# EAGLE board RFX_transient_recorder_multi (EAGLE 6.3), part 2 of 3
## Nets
+2.5V: C18.+ C22.2 C23.2 U5.5 U6.2 U6.44
+2.5V1: C64.+ C65.2 C66.2 U1.2 U1.44 U21.5
+2.5V2: C106.+ C107.2 C108.2 U25.2 U25.44 U33.5
+2.5V3: C148.+ C149.2 C150.2 U37.2 U37.44 U45.5
+2.5V_DIG: C29.2 C30.+ U6.19 U8.5
+2.5V_DIG1: C69.+ C70.2 U1.19 U22.5
+2.5V_DIG2: C111.+ C112.2 U25.19 U34.5
+2.5V_DIG3: C153.+ C154.2 U37.19 U46.5
+3.0V: C14.2 C15.2 C16.+ IC2.8 U4.5 U$1.5 U$1.6 U$1.7 U$1.8
+3.0V1: C50.2 C52.+ C71.2 IC4.8 U20.5 U$2.5 U$2.6 U$2.7 U$2.8
+3.0V2: C92.2 C94.+ C113.2 IC6.8 U32.5 U$3.5 U$3.6 U$3.7 U$3.8
+3.0V3: C134.2 C136.+ C155.2 IC8.8 U44.5 U$4.5 U$4.6 U$4.7 U$4.8
+3V1: C67.+ C68.2 C73.2 C77.2 C78.2 U1.3 U1.4 U1.6 U1.16 U1.18 U2.7 U2.8 U3.1 U16.8 U23.5
+3V2: C109.+ C110.2 C115.2 C119.2 C120.2 U25.3 U25.4 U25.6 U25.16 U25.18 U26.7 U26.8 U27.1 U28.8 U35.5
+3V3: C27.+ C28.2 C32.2 C33.2 C34.2 U6.3 U6.4 U6.6 U6.16 U6.18 U7.5 U9.7 U9.8 U11.1 U12.8
+3V3_ISOL: C35.1 C36.1 C38.+ C41.2 C42.2 R26.2 U11.8 U12.1 U15.4 U15.8
+3V3_ISOL1: C75.1 C76.1 C79.2 C80.2 C84.+ R53.2 U3.8 U16.1 U17.4 U17.8
+3V3_ISOL2: C117.1 C118.1 C121.2 C122.2 C126.+ R81.2 U27.8 U28.1 U29.4 U29.8
+3V3_ISOL3: C159.1 C160.1 C163.2 C164.2 C168.+ R109.2 U39.8 U40.1 U41.4 U41.8
+3V4: C151.+ C152.2 C157.2 C161.2 C162.2 U37.3 U37.4 U37.6 U37.16 U37.18 U38.7 U38.8 U39.1 U40.8 U47.5
+5V_ISOL: C37.+ U10.P$1 U13.1 U13.3
+5V_ISOL1: C83.+ U19.1 U19.3 U24.P$1
+5V_ISOL2: C125.+ U31.1 U31.3 U36.P$1
+5V_ISOL3: C167.+ U43.1 U43.3 U48.P$1
-2.0V_NEG: C4.1 C5.- C6.2 C7.2 IC1.5 IC2.4 R5.2 U$1.13 U$1.14 U$1.15 U$1.16
-2.0V_NEG1: C51.2 C53.- C58.1 C60.2 IC3.5 IC4.4 R33.2 U$2.13 U$2.14 U$2.15 U$2.16
-2.0V_NEG2: C93.2 C95.- C100.1 C102.2 IC5.5 IC6.4 R61.2 U$3.13 U$3.14 U$3.15 U$3.16
-2.0V_NEG3: C135.2 C137.- C142.1 C144.2 IC7.5 IC8.4 R89.2 U$4.13 U$4.14 U$4.15 U$4.16
AGND: C4.2 C5.+ C6.1 C7.1 C11.1 C12.1 C13.2 C14.1 C15.1 C16.- C17.2 C18.- C19.2 C20.- C21.2 C22.1 C23.1 C43.1 IC1.1 IC2.3 R4.2 R17..2 R28.2 U4.2 U5.2 U6.1 U6.36 U6.38 U6.41 U6.42 U6.47 U6.48 X1.1 X1.2 X1.5 X1.6 X2.1 X2.2 X2.5 X2.6 X3.1 X3.2 X3.5 X3.6 X4.1 X4.2 X4.5 X4.6
AGND1: C47.1 C48.1 C49.1 C50.1 C51.1 C52.- C53.+ C54.2 C55.2 C58.2 C60.1 C61.2 C62.- C63.2 C64.- C65.1 C66.1 C71.1 IC3.1 IC4.3 R17.1.2 R32.2 R55.2 U1.1 U1.36 U1.38 U1.41 U1.42 U1.47 U1.48 U20.2 U21.2 X6.1 X6.2 X6.5 X6.6
AGND2: C89.1 C90.1 C91.1 C92.1 C93.1 C94.- C95.+ C96.2 C97.2 C100.2 C102.1 C103.2 C104.- C105.2 C106.- C107.1 C108.1 C113.1 IC5.1 IC6.3 R17.2.2 R60.2 R83.2 U25.1 U25.36 U25.38 U25.41 U25.42 U25.47 U25.48 U32.2 U33.2 X8.1 X8.2 X8.5 X8.6
AGND3: C131.1 C132.1 C133.1 C134.1 C135.1 C136.- C137.+ C138.2 C139.2 C142.2 C144.1 C145.2 C146.- C147.2 C148.- C149.1 C150.1 C155.1 IC7.1 IC8.3 R17.3.2 R88.2 R111.2 U37.1 U37.36 U37.38 U37.41 U37.42 U37.47 U37.48 U44.2 U45.2 X10.1 X10.2 X10.5 X10.6
GNDI: C2..+ C24.1 C25.- C26.2 C27.- C28.1 C29.1 C30.- C31.2 C32.1 C33.1 C34.1 R17..1 R22.1 U6.5 U6.7 U6.13 U6.14 U6.15 U6.17 U6.20 U6.30 U6.31 U6.32 U6.33 U7.2 U8.2 U9.4 U10.P$5 U11.4 U12.5
GNDI1: C2.1.+ C56.2 C57.2 C59.- C67.- C68.1 C69.- C70.1 C73.1 C74.1 C77.1 C78.1 R17.1.1 R56.1 U1.5 U1.7 U1.13 U1.14 U1.15 U1.17 U1.20 U1.30 U1.31 U1.32 U1.33 U2.4 U3.4 U16.5 U22.2 U23.2 U24.P$5
GNDI2: C2.2.+ C98.2 C99.2 C101.- C109.- C110.1 C111.- C112.1 C115.1 C116.1 C119.1 C120.1 R17.2.1 R84.1 U25.5 U25.7 U25.13 U25.14 U25.15 U25.17 U25.20 U25.30 U25.31 U25.32 U25.33 U26.4 U27.4 U28.5 U34.2 U35.2 U36.P$5
GNDI3: C2.3.+ C140.2 C141.2 C143.- C151.- C152.1 C153.- C154.1 C157.1 C158.1 C161.1 C162.1 R17.3.1 R112.1 U37.5 U37.7 U37.13 U37.14 U37.15 U37.17 U37.20 U37.30 U37.31 U37.32 U37.33 U38.4 U39.4 U40.5 U46.2 U47.2 U48.P$5
ISOL_GND: C35.2 C36.2 C37.- C38.- C39.1 C40.1 C41.1 C42.1 R25.2 U10.P$2 U11.5 U12.4 U13.2 U14.4 U15.1 U15.2 U15.3 U15.6 U15.10
ISOL_GND1: C75.2 C76.2 C79.1 C80.1 C81.1 C82.1 C83.- C84.- R54.2 U3.5 U16.4 U17.1 U17.2 U17.3 U17.6 U17.10 U18.4 U19.2 U24.P$2
ISOL_GND2: C117.2 C118.2 C121.1 C122.1 C123.1 C124.1 C125.- C126.- R82.2 U27.5 U28.4 U29.1 U29.2 U29.3 U29.6 U29.10 U30.4 U31.2 U36.P$2
ISOL_GND3: C159.2 C160.2 C163.1 C164.1 C165.1 C166.1 C167.- C168.- R110.2 U39.5 U40.4 U41.1 U41.2 U41.3 U41.6 U41.10 U42.4 U43.2 U48.P$2
N$1: C3.1 L1.2 R6.2
N$2: C1.1 L1.1 R2.1
N$3: C3.2 L2.2 R7.2
N$4: C1.2 L2.1 R3.1
N$5: C9.1 R6.1 R9.1 R11.2 U$1.11
N$6: C10.1 R7.1 R8.1 R12.2 U$1.2
N$7: R20.2 U9.1
N$8: R1.2 R2.2 X1.3
N$9: R1.1 R3.2 X1.4
N$10: C9.2 R11.1 R14.2 U$1.10
N$11: C10.2 R12.1 R15.2 U$1.3
N$12: C11.2 R14.1 U6.39
N$13: C12.2 R15.1 U6.43
N$14: R28.1
N$15: R22.2
N$16: C2..- IC1.2 IC1.3 U10.P$7 X1.9 X1.10
N$17: C17.1 U4.4
N$18: C25.+ U4.1 U4.3 U5.1 U5.3 U7.1 U7.3 U8.1 U8.3 U10.P$6 X1.7 X1.8
N$19: X2.3
N$20: C19.1 U5.4
N$21: X2.4
N$22: X2.9 X2.10 X3.9 X3.10 X4.10
N$23: C31.1 U8.4
N$24: X2.7 X2.8 X3.7 X3.8 X4.7 X4.8
N$25: X3.3
N$26: C26.1 U7.4
N$27: IC1.4 R4.1 R5.1
N$28: C43.2 IC2.6 IC2.7 U$1.4 U$1.9
N$29: X3.4
N$30: C13.1 IC2.5 R13.1 R16.2
N$31: R20.1 U6.22
N$32: C20.+ R16.1 U6.37
N$33: C21.1 U6.46
N$34: U15.11 X5.1
N$35: U15.12 X5.2
N$36: R19.1 U6.23
N$37: R18.2 R19.2 U9.6
N$38: R18.1 U6.29
N$39: U9.2 U9.3
N$40: C8.1 IC2.1 R8.2 R9.2 R10.2
N$41: C8.2 IC2.2 R10.1 R13.2
N$42: U9.5 U11.2
N$43: R21.1 U6.21
N$44: R21.2 U11.3
N$45: C24.2 R17.2 U6.35
N$46: R17.1 U12.6
N$47: U6.34 U12.7
N$48: X4.3
N$49: X4.4
N$50: R27.1 U12.3 U14.1
N$51: R24.2 U15.5
N$52: R23.2 U15.7
N$53: R24.1 U11.7
N$54: R23.1 U11.6
N$55: U15.13 X5.3
N$56: R27.2 U15.9
N$57: R26.1 U12.2 X5.8
N$58: U15.14 X5.4
N$59: U14.2 U14.3
N$60: R25.1 U14.6 X5.7
N$61: U10.P$14 U14.5
N$62: C40.2 U13.5 U14.7 U14.8
N$63: U15.15 X5.5
N$64: C39.2 U13.4
N$65: U15.16 X5.6
N$66: C44.1 L3.2 R34.2
N$67: C2.1 L3.1 R30.1
N$68: C44.2 L4.2 R35.2
N$69: C2.2 L4.1 R31.1
N$70: C45.1 R34.1 R37.1 R38.2 U$2.11
N$71: C46.1 R35.1 R36.1 R39.2 U$2.2
N$72: R29.2 R30.2 X6.3
N$73: R29.1 R31.2 X6.4
N$74: C45.2 R38.1 R40.2 U$2.10
N$75: C46.2 R39.1 R41.2 U$2.3
N$76: C47.2 R40.1 U1.39
N$77: C48.2 R41.1 U1.43
N$78: IC3.4 R32.1 R33.1
N$79: C49.2 IC4.6 IC4.7 U$2.4 U$2.9
N$80: C61.1 IC4.5 R42.2 R43.1
N$81: C62.+ R42.1 U1.37
N$82: C63.1 U1.46
N$83: C72.1 IC4.1 R36.2 R37.2 R44.2
N$84: C72.2 IC4.2 R43.2 R44.1
N$85: R45.2 U2.1
N$86: R45.1 U1.22
N$87: R46.1 U1.23
N$88: R46.2 R47.2 U2.6
N$89: R47.1 U1.29
N$90: U2.2 U2.3
N$91: U2.5 U3.2
N$92: R48.1 U1.21
N$93: R48.2 U3.3
N$94: C74.2 R49.2 U1.35
N$95: R49.1 U16.6
N$96: U1.34 U16.7
N$97: R50.2 U17.5
N$98: R51.2 U17.7
N$99: R50.1 U3.7
N$100: R51.1 U3.6
N$101: R52.2 U17.9
N$102: R52.1 U16.3 U18.1
N$103: R53.1 U16.2 X7.8
N$104: U18.2 U18.3
N$105: R54.1 U18.6 X7.7
N$106: C81.2 U18.7 U18.8 U19.5
N$107: C82.2 U19.4
N$108: C54.1 U20.4
N$109: C55.1 U21.4
N$110: C56.1 U22.4
N$111: C57.1 U23.4
N$112: U18.5 U24.P$14
N$113: R55.1
N$114: R56.2
N$115: C2.1.- IC3.2 IC3.3 U24.P$7 X6.9 X6.10
N$116: C59.+ U20.1 U20.3 U21.1 U21.3 U22.1 U22.3 U23.1 U23.3 U24.P$6 X6.7 X6.8
N$117: U17.11 X7.1
N$118: U17.12 X7.2
N$119: U17.13 X7.3
N$120: U17.14 X7.4
N$121: U17.15 X7.5
N$122: U17.16 X7.6
N$123: C86.1 L5.2 R62.2
N$124: C85.1 L5.1 R58.1
N$125: C86.2 L6.2 R63.2
N$126: C85.2 L6.1 R59.1
N$127: C87.1 R62.1 R65.1 R66.2 U$3.11
N$128: C88.1 R63.1 R64.1 R67.2 U$3.2
N$129: R57.2 R58.2 X8.3
N$130: R57.1 R59.2 X8.4
N$131: C87.2 R66.1 R68.2 U$3.10
N$132: C88.2 R67.1 R69.2 U$3.3
N$133: C89.2 R68.1 U25.39
N$134: C90.2 R69.1 U25.43
N$135: IC5.4 R60.1 R61.1
N$136: C91.2 IC6.6 IC6.7 U$3.4 U$3.9
N$137: C103.1 IC6.5 R70.2 R71.1
N$138: C104.+ R70.1 U25.37
N$139: C105.1 U25.46
N$140: C114.1 IC6.1 R64.2 R65.2 R72.2
N$141: C114.2 IC6.2 R71.2 R72.1
N$142: R73.2 U26.1
N$143: R73.1 U25.22
N$144: R74.1 U25.23
N$145: R74.2 R75.2 U26.6
N$146: R75.1 U25.29
N$147: U26.2 U26.3
N$148: U26.5 U27.2
N$149: R76.1 U25.21
N$150: R76.2 U27.3
N$151: C116.2 R77.2 U25.35
N$152: R77.1 U28.6
N$153: U25.34 U28.7
N$154: R78.2 U29.5
N$155: R79.2 U29.7
N$156: R78.1 U27.7
N$157: R79.1 U27.6
N$158: R80.2 U29.9
N$159: R80.1 U28.3 U30.1
N$160: R81.1 U28.2 X9.8
N$161: U30.2 U30.3
N$162: R82.1 U30.6 X9.7
N$163: C123.2 U30.7 U30.8 U31.5
N$164: C124.2 U31.4
N$165: C96.1 U32.4
N$166: C97.1 U33.4
N$167: C98.1 U34.4
N$168: C99.1 U35.4
N$169: U30.5 U36.P$14
N$170: R83.1
N$171: R84.2
N$172: C2.2.- IC5.2 IC5.3 U36.P$7 X8.9 X8.10
N$173: C101.+ U32.1 U32.3 U33.1 U33.3 U34.1 U34.3 U35.1 U35.3 U36.P$6 X8.7 X8.8
N$174: U29.11 X9.1
N$175: U29.12 X9.2
N$176: U29.13 X9.3
N$177: U29.14 X9.4
N$178: U29.15 X9.5
N$179: U29.16 X9.6
N$180: C128.1 L7.2 R90.2
N$181: C127.1 L7.1 R86.1
N$182: C128.2 L8.2 R91.2
N$183: C127.2 L8.1 R87.1
N$184: C129.1 R90.1 R93.1 R94.2 U$4.11
N$185: C130.1 R91.1 R92.1 R95.2 U$4.2
N$186: R85.2 R86.2 X10.3
N$187: R85.1 R87.2 X10.4
N$188: C129.2 R94.1 R96.2 U$4.10
N$189: C130.2 R95.1 R97.2 U$4.3
N$190: C131.2 R96.1 U37.39
N$191: C132.2 R97.1 U37.43
N$192: IC7.4 R88.1 R89.1
N$193: C133.2 IC8.6 IC8.7 U$4.4 U$4.9
N$194: C145.1 IC8.5 R98.2 R99.1
N$195: C146.+ R98.1 U37.37
N$196: C147.1 U37.46
N$197: C156.1 IC8.1 R92.2 R93.2 R100.2
N$198: C156.2 IC8.2 R99.2 R100.1
N$199: R101.2 U38.1
N$200: R101.1 U37.22
N$201: R102.1 U37.23
N$202: R102.2 R103.2 U38.6
N$203: R103.1 U37.29
N$204: U38.2 U38.3
N$205: U38.5 U39.2
N$206: R104.1 U37.21
N$207: R104.2 U39.3
N$208: C158.2 R105.2 U37.35
N$209: R105.1 U40.6
N$210: U37.34 U40.7
N$211: R106.2 U41.5
N$212: R107.2 U41.7
N$213: R106.1 U39.7
N$214: R107.1 U39.6
N$215: R108.2 U41.9
N$216: R108.1 U40.3 U42.1
N$217: R109.1 U40.2 X11.8
N$218: U42.2 U42.3
N$219: R110.1 U42.6 X11.7
N$220: C165.2 U42.7 U42.8 U43.5
N$221: C166.2 U43.4
N$222: C138.1 U44.4
N$223: C139.1 U45.4
N$224: C140.1 U46.4
N$225: C141.1 U47.4
N$226: U42.5 U48.P$14
N$227: R111.1
N$228: R112.2
N$229: C2.3.- IC7.2 IC7.3 U48.P$7 X10.9 X10.10
N$230: C143.+ U44.1 U44.3 U45.1 U45.3 U46.1 U46.3 U47.1 U47.3 U48.P$6 X10.7 X10.8
N$231: U41.11 X11.1
N$232: U41.12 X11.2
N$233: U41.13 X11.3
N$234: U41.14 X11.4
N$235: U41.15 X11.5
N$236: U41.16 X11.6

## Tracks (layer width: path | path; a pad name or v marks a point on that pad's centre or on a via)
+2.5V
  Top 0.254: 55.9,84.53 56.5,84.53 56.5,83.93 C23.2 56.5,83.73 56.5,81.33 C22.2 56.6,81.23 57.4,80.43 57.4,74.33 | 55.9,84.53 51.1,84.53 U6.44 | 55.9,84.53 55.9,86.83 55.7,87.03 55.7,88.83 49.5,88.83 49.3,88.63 49.3,87.93 U6.2 | 57.4,74.33 61.4,74.33 62.2,75.13 62.2,76.53 U5.5 | C18.+ 43,76.13 44.9,74.23 57.3,74.23 57.3,74.33 57.4,74.33
+2.5V1
  Top 0.254: 55.9,12.14 56.5,12.14 56.5,11.54 C66.2 56.5,11.34 56.5,8.94 C65.2 56.6,8.84 57.4,8.04 57.4,1.94 | 55.9,12.14 51.1,12.14 U1.44 | 55.9,12.14 55.9,14.44 55.7,14.64 55.7,16.44 49.5,16.44 49.3,16.24 49.3,15.54 U1.2 | 57.4,1.94 61.4,1.94 62.2,2.74 62.2,4.14 U21.5 | C64.+ 43,3.74 44.9,1.84 57.3,1.84 57.3,1.94 57.4,1.94
+2.5V2
  Top 0.254: 55.9,60.4 56.5,60.4 56.5,59.8 C108.2 56.5,59.6 56.5,57.2 C107.2 56.6,57.1 57.4,56.3 57.4,50.2 | 55.9,60.4 51.1,60.4 U25.44 | 55.9,60.4 55.9,62.7 55.7,62.9 55.7,64.7 49.5,64.7 49.3,64.5 49.3,63.8 U25.2 | 57.4,50.2 61.4,50.2 62.2,51 62.2,52.4 U33.5 | C106.+ 43,52 44.9,50.1 57.3,50.1 57.3,50.2 57.4,50.2
+2.5V3
  Top 0.254: 55.9,36.27 56.5,36.27 56.5,35.67 C150.2 56.5,35.47 56.5,33.07 C149.2 56.6,32.97 57.4,32.17 57.4,26.07 | 55.9,36.27 51.1,36.27 U37.44 | 55.9,36.27 55.9,38.57 55.7,38.77 55.7,40.57 49.5,40.57 49.3,40.37 49.3,39.67 U37.2 | 57.4,26.07 61.4,26.07 62.2,26.87 62.2,28.27 U45.5 | C148.+ 43,27.87 44.9,25.97 57.3,25.97 57.3,26.07 57.4,26.07
+2.5V_DIG
  Top 0.254: 38.7,95.53 38.7,95.63 37.9,96.43 C30.+ | 38.7,95.53 38.7,91.53 C29.2 38.8,91.33 39.4,90.73 39.4,86.53 41.4,84.53 41.4,83.63 42.8,83.63 U6.19 | 38.7,95.53 49.1,95.53 49.7,96.13 49.7,97.93 60.7,97.93 60.9,97.73 60.9,95.63 64.7,95.63 U8.5
+2.5V_DIG1
  Top 0.254: 38.7,23.14 38.7,23.24 37.9,24.04 C69.+ | 38.7,23.14 38.7,19.14 C70.2 38.8,18.94 39.4,18.34 39.4,14.14 41.4,12.14 41.4,11.24 42.8,11.24 U1.19 | 38.7,23.14 49.1,23.14 49.7,23.74 49.7,25.54 60.7,25.54 60.9,25.34 60.9,23.24 64.7,23.24 U22.5
+2.5V_DIG2
  Top 0.254: 38.7,71.4 38.7,71.5 37.9,72.3 C111.+ | 38.7,71.4 38.7,67.4 C112.2 38.8,67.2 39.4,66.6 39.4,62.4 41.4,60.4 41.4,59.5 42.8,59.5 U25.19 | 38.7,71.4 49.1,71.4 49.7,72 49.7,73.8 60.7,73.8 60.9,73.6 60.9,71.5 64.7,71.5 U34.5
+2.5V_DIG3
  Top 0.254: 38.7,47.27 38.7,47.37 37.9,48.17 C153.+ | 38.7,47.27 38.7,43.27 C154.2 38.8,43.07 39.4,42.47 39.4,38.27 41.4,36.27 41.4,35.37 42.8,35.37 U37.19 | 38.7,47.27 49.1,47.27 49.7,47.87 49.7,49.67 60.7,49.67 60.9,49.47 60.9,47.37 64.7,47.37 U46.5
+3.0V  (via drill 0.61, 0.61 layers 1-2)
  Top 0.254: U$1.8 19.6,85.33 20,85.33 U$1.7 20.1,85.33 20.5,85.33 U$1.6 20.6,85.33 21,85.33 U$1.5 21,85.43 21.1,85.53 21.1,85.63 21.6,86.13 23,86.13 | C16.+ 21.8,77.53 21.8,79.13 21,79.93 C15.2 21,80.13 21,81.13 v20.8,81.33 | v23,84.83 23,86.13 | U4.5 64.7,90.43 64.7,88.93 61.7,88.93 C14.2 61.6,89.03 61.6,91.93 v60.4,93.13 | v57.2,94.33 57.2,94.93 | 57.2,94.93 57.2,95.93 56.6,96.53 IC2.8 | v37.9,94.63 36.8,95.73 36.8,97.23 30.6,97.23 29.7,96.33 29.7,92.93 23,86.23 23,86.13 | v39.5,94.63 45.7,94.63 45.7,94.83 45.8,94.93 57.2,94.93
  top_internal 0.254: v57.2,94.33 58.4,93.13 v60.4,93.13 | v39.5,94.63 v37.9,94.63
  bottom_internal 0.254: v23,84.83 20.8,82.63 v20.8,81.33
+3.0V1  (via drill 0.61, 0.61 layers 1-2)
  Top 0.254: U$2.8 19.6,12.94 20,12.94 U$2.7 20.1,12.94 20.5,12.94 U$2.6 20.6,12.94 21,12.94 U$2.5 21,13.04 21.1,13.14 21.1,13.24 21.6,13.74 23,13.74 | C52.+ 21.8,5.14 21.8,6.74 21,7.54 C50.2 21,7.74 21,8.74 v20.8,8.94 | v23,12.44 23,13.74 | U20.5 64.7,18.04 64.7,16.54 61.7,16.54 C71.2 61.6,16.64 61.6,19.54 v60.4,20.74 | v57.2,21.94 57.2,22.54 | 57.2,22.54 57.2,23.54 56.6,24.14 IC4.8 | v37.9,22.24 36.8,23.34 36.8,24.84 30.6,24.84 29.7,23.94 29.7,20.54 23,13.84 23,13.74 | v39.5,22.24 45.7,22.24 45.7,22.44 45.8,22.54 57.2,22.54
  top_internal 0.254: v57.2,21.94 58.4,20.74 v60.4,20.74 | v39.5,22.24 v37.9,22.24
  bottom_internal 0.254: v23,12.44 20.8,10.24 v20.8,8.94
+3.0V2  (via drill 0.61, 0.61 layers 1-2)
  Top 0.254: U$3.8 19.6,61.2 20,61.2 U$3.7 20.1,61.2 20.5,61.2 U$3.6 20.6,61.2 21,61.2 U$3.5 21,61.3 21.1,61.4 21.1,61.5 21.6,62 23,62 | C94.+ 21.8,53.4 21.8,55 21,55.8 C92.2 21,56 21,57 v20.8,57.2 | v23,60.7 23,62 | U32.5 64.7,66.3 64.7,64.8 61.7,64.8 C113.2 61.6,64.9 61.6,67.8 v60.4,69 | v57.2,70.2 57.2,70.8 | 57.2,70.8 57.2,71.8 56.6,72.4 IC6.8 | v37.9,70.5 36.8,71.6 36.8,73.1 30.6,73.1 29.7,72.2 29.7,68.8 23,62.1 23,62 | v39.5,70.5 45.7,70.5 45.7,70.7 45.8,70.8 57.2,70.8
  top_internal 0.254: v57.2,70.2 58.4,69 v60.4,69 | v39.5,70.5 v37.9,70.5
  bottom_internal 0.254: v23,60.7 20.8,58.5 v20.8,57.2
+3.0V3  (via drill 0.61, 0.61 layers 1-2)
  Top 0.254: U$4.8 19.6,37.07 20,37.07 U$4.7 20.1,37.07 20.5,37.07 U$4.6 20.6,37.07 21,37.07 U$4.5 21,37.17 21.1,37.27 21.1,37.37 21.6,37.87 23,37.87 | C136.+ 21.8,29.27 21.8,30.87 21,31.67 C134.2 21,31.87 21,32.87 v20.8,33.07 | v23,36.57 23,37.87 | U44.5 64.7,42.17 64.7,40.67 61.7,40.67 C155.2 61.6,40.77 61.6,43.67 v60.4,44.87 | v57.2,46.07 57.2,46.67 | 57.2,46.67 57.2,47.67 56.6,48.27 IC8.8 | v37.9,46.37 36.8,47.47 36.8,48.97 30.6,48.97 29.7,48.07 29.7,44.67 23,37.97 23,37.87 | v39.5,46.37 45.7,46.37 45.7,46.57 45.8,46.67 57.2,46.67
  top_internal 0.254: v57.2,46.07 58.4,44.87 v60.4,44.87 | v39.5,46.37 v37.9,46.37
  bottom_internal 0.254: v23,36.57 20.8,34.37 v20.8,33.07
+3V1  (via drill 0.61, 0.61 layers 1-2)
  Top 0.254: U2.8 29.9,8.94 31,8.94 U2.7 31.2,9.04 31.2,10.14 31.7,10.64 31.7,14.44 32.5,15.24 C73.2 37.5,15.14 39.8,12.84 v39.8,12.64 | 42,12.44 42,11.74 42.8,11.74 U1.18 | 42,12.44 42.2,12.64 42.8,12.64 U1.16 43,12.74 47.2,12.74 47.2,15.44 U1.6 47.3,15.54 47.3,16.24 48.7,17.64 48.8,17.64 | 48.8,17.44 48.8,15.54 U1.3 48.7,15.54 48.3,15.54 U1.4 | 48.8,17.44 48.8,17.64 | 48.8,17.64 48.8,18.94 C68.2 48.9,19.14 48.9,20.74 49.7,21.54 C67.+ | v40.9,13.74 42,12.64 42,12.44 | U16.8 90.2,3.24 91.5,3.24 91.5,13.74 90.7,14.54 90.2,14.54 U3.1 90,14.64 79.3,14.64 | 75.3,14.04 79.3,14.04 79.3,14.64 | 75.3,14.04 74.4,14.04 C78.2 | 79.3,14.64 79.3,16.44 C77.2 | v67.7,6.34 67.7,4.54 66.1,2.94 U23.5 | v75.3,13.94 75.3,14.04 | v55.7,17.44 48.8,17.44
  top_internal 0.254: v40.9,13.74 v39.8,12.64
  bottom_internal 0.254: v75.3,13.94 v67.7,6.34
  Bottom 0.254: v55.7,17.44 66.8,6.34 v67.7,6.34
+3V2  (via drill 0.61, 0.61 layers 1-2)
  Top 0.254: U26.8 29.9,57.2 31,57.2 U26.7 31.2,57.3 31.2,58.4 31.7,58.9 31.7,62.7 32.5,63.5 C115.2 37.5,63.4 39.8,61.1 v39.8,60.9 | 42,60.7 42,60 42.8,60 U25.18 | 42,60.7 42.2,60.9 42.8,60.9 U25.16 43,61 47.2,61 47.2,63.7 U25.6 47.3,63.8 47.3,64.5 48.7,65.9 48.8,65.9 | 48.8,65.7 48.8,63.8 U25.3 48.7,63.8 48.3,63.8 U25.4 | 48.8,65.7 48.8,65.9 | 48.8,65.9 48.8,67.2 C110.2 48.9,67.4 48.9,69 49.7,69.8 C109.+ | v40.9,62 42,60.9 42,60.7 | U28.8 90.2,51.5 91.5,51.5 91.5,62 90.7,62.8 90.2,62.8 U27.1 90,62.9 79.3,62.9 | 75.3,62.3 79.3,62.3 79.3,62.9 | 75.3,62.3 74.4,62.3 C120.2 | 79.3,62.9 79.3,64.7 C119.2 | v67.7,54.6 67.7,52.8 66.1,51.2 U35.5 | v75.3,62.2 75.3,62.3 | v55.7,65.7 48.8,65.7
  top_internal 0.254: v40.9,62 v39.8,60.9
  bottom_internal 0.254: v75.3,62.2 v67.7,54.6
  Bottom 0.254: v55.7,65.7 66.8,54.6 v67.7,54.6
+3V3  (via drill 0.61, 0.61 layers 1-2)
  Top 0.254: U9.8 29.9,81.33 31,81.33 U9.7 31.2,81.43 31.2,82.53 31.7,83.03 31.7,86.83 32.5,87.63 C32.2 37.5,87.53 39.8,85.23 v39.8,85.03 | 42,84.83 42,84.13 42.8,84.13 U6.18 | 42,84.83 42.2,85.03 42.8,85.03 U6.16 43,85.13 47.2,85.13 47.2,87.83 U6.6 47.3,87.93 47.3,88.63 48.7,90.03 48.8,90.03 | 48.8,89.83 48.8,87.93 U6.3 48.7,87.93 48.3,87.93 U6.4 | 48.8,89.83 48.8,90.03 | 48.8,90.03 48.8,91.33 C28.2 48.9,91.53 48.9,93.13 49.7,93.93 C27.+ | v40.9,86.13 42,85.03 42,84.83 | U12.8 90.2,75.63 91.5,75.63 91.5,86.13 90.7,86.93 90.2,86.93 U11.1 90,87.03 79.3,87.03 | 75.3,86.43 79.3,86.43 79.3,87.03 | 75.3,86.43 74.4,86.43 C33.2 | 79.3,87.03 79.3,88.83 C34.2 | v67.7,78.73 67.7,76.93 66.1,75.33 U7.5 | v75.3,86.33 75.3,86.43 | v55.7,89.83 48.8,89.83
  top_internal 0.254: v40.9,86.13 v39.8,85.03
  bottom_internal 0.254: v75.3,86.33 v67.7,78.73
  Bottom 0.254: v55.7,89.83 66.8,78.73 v67.7,78.73
+3V3_ISOL
  Top 0.254: 109.9,92.73 109.9,93.93 C35.1 | 109.9,92.73 109.9,91.53 C36.1 109.8,91.33 109,90.53 109,81.73 106.6,79.33 106.6,79.23 | 109.9,92.73 116.1,92.73 C42.2 116.2,92.63 116.2,77.53 C41.2 | 106.6,79.23 107.1,78.73 107.1,76.53 105.1,76.53 U15.8 104.9,76.43 104.5,76.43 104.1,76.03 104.1,75.63 97.6,75.63 | 106.6,79.23 105.1,79.23 105.1,79.13 U15.4 | 97.6,75.63 95.4,75.63 U12.1 | C38.+ 105.6,93.93 104.7,93.93 102.3,91.53 R26.2 102.2,91.33 97.9,87.03 97.6,87.03 | 97.6,87.03 95.4,87.03 U11.8 | 97.6,87.03 97.6,75.63
+3V3_ISOL1
  Top 0.254: 109.9,20.34 109.9,21.54 C76.1 | 109.9,20.34 109.9,19.14 C75.1 109.8,18.94 109,18.14 109,9.34 106.6,6.94 106.6,6.84 | 109.9,20.34 116.1,20.34 C79.2 116.2,20.24 116.2,5.14 C80.2 | 106.6,6.84 107.1,6.34 107.1,4.14 105.1,4.14 U17.8 104.9,4.04 104.5,4.04 104.1,3.64 104.1,3.24 97.6,3.24 | 106.6,6.84 105.1,6.84 105.1,6.74 U17.4 | 97.6,3.24 95.4,3.24 U16.1 | C84.+ 105.6,21.54 104.7,21.54 102.3,19.14 R53.2 102.2,18.94 97.9,14.64 97.6,14.64 | 97.6,14.64 95.4,14.64 U3.8 | 97.6,14.64 97.6,3.24
+3V3_ISOL2
  Top 0.254: 109.9,68.6 109.9,69.8 C118.1 | 109.9,68.6 109.9,67.4 C117.1 109.8,67.2 109,66.4 109,57.6 106.6,55.2 106.6,55.1 | 109.9,68.6 116.1,68.6 C121.2 116.2,68.5 116.2,53.4 C122.2 | 106.6,55.1 107.1,54.6 107.1,52.4 105.1,52.4 U29.8 104.9,52.3 104.5,52.3 104.1,51.9 104.1,51.5 97.6,51.5 | 106.6,55.1 105.1,55.1 105.1,55 U29.4 | 97.6,51.5 95.4,51.5 U28.1 | C126.+ 105.6,69.8 104.7,69.8 102.3,67.4 R81.2 102.2,67.2 97.9,62.9 97.6,62.9 | 97.6,62.9 95.4,62.9 U27.8 | 97.6,62.9 97.6,51.5
+3V3_ISOL3
  Top 0.254: 109.9,44.47 109.9,45.67 C160.1 | 109.9,44.47 109.9,43.27 C159.1 109.8,43.07 109,42.27 109,33.47 106.6,31.07 106.6,30.97 | 109.9,44.47 116.1,44.47 C163.2 116.2,44.37 116.2,29.27 C164.2 | 106.6,30.97 107.1,30.47 107.1,28.27 105.1,28.27 U41.8 104.9,28.17 104.5,28.17 104.1,27.77 104.1,27.37 97.6,27.37 | 106.6,30.97 105.1,30.97 105.1,30.87 U41.4 | 97.6,27.37 95.4,27.37 U40.1 | C168.+ 105.6,45.67 104.7,45.67 102.3,43.27 R109.2 102.2,43.07 97.9,38.77 97.6,38.77 | 97.6,38.77 95.4,38.77 U39.8 | 97.6,38.77 97.6,27.37
+3V4  (via drill 0.61, 0.61 layers 1-2)
  Top 0.254: U38.8 29.9,33.07 31,33.07 U38.7 31.2,33.17 31.2,34.27 31.7,34.77 31.7,38.57 32.5,39.37 C157.2 37.5,39.27 39.8,36.97 v39.8,36.77 | 42,36.57 42,35.87 42.8,35.87 U37.18 | 42,36.57 42.2,36.77 42.8,36.77 U37.16 43,36.87 47.2,36.87 47.2,39.57 U37.6 47.3,39.67 47.3,40.37 48.7,41.77 48.8,41.77 | 48.8,41.57 48.8,39.67 U37.3 48.7,39.67 48.3,39.67 U37.4 | 48.8,41.57 48.8,41.77 | 48.8,41.77 48.8,43.07 C152.2 48.9,43.27 48.9,44.87 49.7,45.67 C151.+ | v40.9,37.87 42,36.77 42,36.57 | U40.8 90.2,27.37 91.5,27.37 91.5,37.87 90.7,38.67 90.2,38.67 U39.1 90,38.77 79.3,38.77 | 75.3,38.17 79.3,38.17 79.3,38.77 | 75.3,38.17 74.4,38.17 C162.2 | 79.3,38.77 79.3,40.57 C161.2 | v67.7,30.47 67.7,28.67 66.1,27.07 U47.5 | v75.3,38.07 75.3,38.17 | v55.7,41.57 48.8,41.57
  top_internal 0.254: v40.9,37.87 v39.8,36.77
  bottom_internal 0.254: v75.3,38.07 v67.7,30.47
  Bottom 0.254: v55.7,41.57 66.8,30.47 v67.7,30.47
+5V_ISOL  (via drill 0.61, 0.61 layers 1-2)
  Top 0.254: v111.1,95.23 112,95.23 U13.1 | v113.6,96.43 113.6,95.53 113.9,95.23 U13.3 | v105.7,96.43 105.7,97.73 C37.+
  top_internal 0.254: v113.6,96.43 112.4,95.23 v111.1,95.23
  bottom_internal 0.254: 105.7,95.23 97.8,95.23 97.8,96.43 U10.P$1 | 105.7,95.23 v111.1,95.23 | 105.7,95.23 v105.7,96.43
+5V_ISOL1  (via drill 0.61, 0.61 layers 1-2)
  Top 0.254: v111.1,22.84 112,22.84 U19.1 | v113.6,24.04 113.6,23.14 113.9,22.84 U19.3 | v105.7,24.04 105.7,25.34 C83.+
  top_internal 0.254: v113.6,24.04 112.4,22.84 v111.1,22.84
  bottom_internal 0.254: 105.7,22.84 97.8,22.84 97.8,24.04 U24.P$1 | 105.7,22.84 v111.1,22.84 | 105.7,22.84 v105.7,24.04
+5V_ISOL2  (via drill 0.61, 0.61 layers 1-2)
  Top 0.254: v111.1,71.1 112,71.1 U31.1 | v113.6,72.3 113.6,71.4 113.9,71.1 U31.3 | v105.7,72.3 105.7,73.6 C125.+
  top_internal 0.254: v113.6,72.3 112.4,71.1 v111.1,71.1
  bottom_internal 0.254: 105.7,71.1 97.8,71.1 97.8,72.3 U36.P$1 | 105.7,71.1 v111.1,71.1 | 105.7,71.1 v105.7,72.3
+5V_ISOL3  (via drill 0.61, 0.61 layers 1-2)
  Top 0.254: v111.1,46.97 112,46.97 U43.1 | v113.6,48.17 113.6,47.27 113.9,46.97 U43.3 | v105.7,48.17 105.7,49.47 C167.+
  top_internal 0.254: v113.6,48.17 112.4,46.97 v111.1,46.97
  bottom_internal 0.254: 105.7,46.97 97.8,46.97 97.8,48.17 U48.P$1 | 105.7,46.97 v111.1,46.97 | 105.7,46.97 v105.7,48.17
-2.0V_NEG  (via drill 0.61 layers 1-2)
  Top 0.254: v70.8,84.43 70.8,83.83 C4.1 | v67.3,85.23 66.1,85.23 66.1,85.33 IC1.5 65.9,85.43 61.6,85.43 | 61.6,85.43 61.6,86.33 R5.2 61.5,86.43 61.5,87.73 61,88.23 61,89.43 60.5,89.93 60.5,91.23 60.4,91.33 IC2.4 | 61.6,85.43 61.6,85.03 61,84.43 61,81.93 61.6,81.33 C6.2 61.5,81.23 59.2,78.93 v59.2,78.43 | U$1.13 19.6,82.33 20,82.33 U$1.14 20.2,82.33 20.5,82.33 U$1.15 20.7,82.33 21,82.33 U$1.16 21.1,82.23 21.4,81.93 21.4,81.83 22.9,81.83 | 22.9,81.83 26.5,81.83 26.7,82.03 26.7,83.93 29.1,86.33 29.1,87.73 30.1,88.73 30.1,95.43 31.1,96.43 C7.2 | 22.9,81.83 22.9,75.93 21.9,74.93 C5.- 21.9,74.83 21.9,74.73 38.5,74.73 39.4,75.63 39.4,77.13 48.3,77.13 49,77.83 v49.9,77.83
  top_internal 0.254: v70.8,84.43 70,85.23 v67.3,85.23 | v59.2,78.43 58.9,78.13 50.2,78.13 v49.9,77.83
-2.0V_NEG1  (via drill 0.61 layers 1-2)
  Top 0.254: v70.8,12.04 70.8,11.44 C58.1 | v67.3,12.84 66.1,12.84 66.1,12.94 IC3.5 65.9,13.04 61.6,13.04 | 61.6,13.04 61.6,13.94 R33.2 61.5,14.04 61.5,15.34 61,15.84 61,17.04 60.5,17.54 60.5,18.84 60.4,18.94 IC4.4 | 61.6,13.04 61.6,12.64 61,12.04 61,9.54 61.6,8.94 C60.2 61.5,8.84 59.2,6.54 v59.2,6.04 | U$2.13 19.6,9.94 20,9.94 U$2.14 20.2,9.94 20.5,9.94 U$2.15 20.7,9.94 21,9.94 U$2.16 21.1,9.84 21.4,9.54 21.4,9.44 22.9,9.44 | 22.9,9.44 26.5,9.44 26.7,9.64 26.7,11.54 29.1,13.94 29.1,15.34 30.1,16.34 30.1,23.04 31.1,24.04 C51.2 | 22.9,9.44 22.9,3.54 21.9,2.54 C53.- 21.9,2.44 21.9,2.34 38.5,2.34 39.4,3.24 39.4,4.74 48.3,4.74 49,5.44 v49.9,5.44
  top_internal 0.254: v70.8,12.04 70,12.84 v67.3,12.84 | v59.2,6.04 58.9,5.74 50.2,5.74 v49.9,5.44
-2.0V_NEG2  (via drill 0.61 layers 1-2)
  Top 0.254: v70.8,60.3 70.8,59.7 C100.1 | v67.3,61.1 66.1,61.1 66.1,61.2 IC5.5 65.9,61.3 61.6,61.3 | 61.6,61.3 61.6,62.2 R61.2 61.5,62.3 61.5,63.6 61,64.1 61,65.3 60.5,65.8 60.5,67.1 60.4,67.2 IC6.4 | 61.6,61.3 61.6,60.9 61,60.3 61,57.8 61.6,57.2 C102.2 61.5,57.1 59.2,54.8 v59.2,54.3 | U$3.13 19.6,58.2 20,58.2 U$3.14 20.2,58.2 20.5,58.2 U$3.15 20.7,58.2 21,58.2 U$3.16 21.1,58.1 21.4,57.8 21.4,57.7 22.9,57.7 | 22.9,57.7 26.5,57.7 26.7,57.9 26.7,59.8 29.1,62.2 29.1,63.6 30.1,64.6 30.1,71.3 31.1,72.3 C93.2 | 22.9,57.7 22.9,51.8 21.9,50.8 C95.- 21.9,50.7 21.9,50.6 38.5,50.6 39.4,51.5 39.4,53 48.3,53 49,53.7 v49.9,53.7
  top_internal 0.254: v70.8,60.3 70,61.1 v67.3,61.1 | v59.2,54.3 58.9,54 50.2,54 v49.9,53.7
-2.0V_NEG3  (via drill 0.61 layers 1-2)
  Top 0.254: v70.8,36.17 70.8,35.57 C142.1 | v67.3,36.97 66.1,36.97 66.1,37.07 IC7.5 65.9,37.17 61.6,37.17 | 61.6,37.17 61.6,38.07 R89.2 61.5,38.17 61.5,39.47 61,39.97 61,41.17 60.5,41.67 60.5,42.97 60.4,43.07 IC8.4 | 61.6,37.17 61.6,36.77 61,36.17 61,33.67 61.6,33.07 C144.2 61.5,32.97 59.2,30.67 v59.2,30.17 | U$4.13 19.6,34.07 20,34.07 U$4.14 20.2,34.07 20.5,34.07 U$4.15 20.7,34.07 21,34.07 U$4.16 21.1,33.97 21.4,33.67 21.4,33.57 22.9,33.57 | 22.9,33.57 26.5,33.57 26.7,33.77 26.7,35.67 29.1,38.07 29.1,39.47 30.1,40.47 30.1,47.17 31.1,48.17 C135.2 | 22.9,33.57 22.9,27.67 21.9,26.67 C137.- 21.9,26.57 21.9,26.47 38.5,26.47 39.4,27.37 39.4,28.87 48.3,28.87 49,29.57 v49.9,29.57
  top_internal 0.254: v70.8,36.17 70,36.97 v67.3,36.97 | v59.2,30.17 58.9,29.87 50.2,29.87 v49.9,29.57
AGND  (via drill 0.61)  (1 unrouted)
  Top 0.254: 14,19.03 14,20.23 X4.2 14,20.43 14,41.83 X3.1 14,41.93 14,43.23 | 14,19.03 14,17.83 X4.1 | 19.1,19.03 19.1,20.23 X4.6 | 19.1,19.03 19.1,17.83 X4.5 | 19.1,19.03 14,19.03 | 14,43.23 14,44.43 X3.2 | 19.1,43.23 19.1,44.43 X3.6 | 19.1,43.23 19.1,41.93 X3.5 | 19.1,43.23 14,43.23 | 14,44.53 X3.2 | 14,44.63 X3.2 | 14,44.73 X3.2 | 14,67.33 14,68.53 X2.2 | 14,67.33 14,66.13 X2.1 14,65.93 14,44.83 X3.2 | 19.1,67.33 19.1,68.53 X2.6 | 19.1,67.33 19.1,66.13 X2.5 | 19.1,67.33 14,67.33 | R28.2 73.1,74.93 v74.2,76.03 74.3,76.13 74.3,77.43 R17..2 74.2,77.53 73.7,78.03 73.7,84.33 73.75,84.38 | 73.75,84.38 73.7,84.43 73.7,88.23 74.3,88.83 R4.2 | 73.75,84.38 C4.2 | 60.3,82.13 60.3,83.73 C13.2 | 60.3,82.13 60.3,81.33 C6.1 | 60.3,82.13 v58.7,82.13 58.7,91.03 59,91.33 IC2.3 | 50.45,87.18 51,86.63 U6.48 51.1,86.53 51.1,86.13 U6.47 51,86.03 50.2,86.03 50.2,83.03 | 50.45,87.18 49.8,87.83 U6.1 | U6.42 51.1,83.53 51.1,83.13 U6.41 51,83.03 50.2,83.03 | 50.2,81.33 50.2,80.13 49.8,79.73 U6.36 | 50.2,81.33 50.4,81.53 51,81.53 U6.38 | 50.2,81.33 50.2,83.03 | U4.2 67.3,91.43 66.5,91.43 v66.5,89.63 66.5,88.03 67.7,86.83 67.7,86.03 68.3,85.43 68.6,85.43 IC1.1 | C15.1 19.6,79.93 18.9,79.23 v18.9,78.83 18.9,77.53 C16.- 18.9,77.43 18.9,74.93 C5.+ | C18.- 46,76.23 v47.7,76.23 49.3,76.23 C20.- | C7.1 v32.4,94.63 C43.1 | 79.4,83.83 79.4,85.03 C19.2 | 79.4,83.83 79.4,82.63 C17.2 | C22.1 55.2,81.33 v55.2,82.53 55.2,83.73 C23.1 | v23.7,80.03 24.7,80.03 C12.1 | v24.8,84.03 24.8,85.03 C11.1 | v56.5,87.43 56.5,86.43 C21.2 | v60.3,87.83 60.3,88.83 C14.1 | v67.4,81.33 68.6,81.33 U5.2 | v79.6,83.83 79.4,83.83 | v50.5,87.33 50.5,87.23 50.45,87.18
  pour Bottom: -1.27,100.33 91.44,100.33 91.44,73.66 0,73.66
  pour bottom_internal: -5.08,104.14 91.44,104.14 90.17,-1.27 -6.35,-1.27
AGND1  (via drill 0.61)  (1 unrouted)
  Top 0.254: R55.2 73.1,2.54 v74.2,3.64 74.3,3.74 74.3,5.04 R17.1.2 74.2,5.14 73.7,5.64 73.7,11.94 73.75,11.99 | 73.75,11.99 73.7,12.04 73.7,15.84 74.3,16.44 R32.2 | 73.75,11.99 C58.2 | 60.3,9.74 60.3,11.34 C61.2 | 60.3,9.74 60.3,8.94 C60.1 | 60.3,9.74 v58.7,9.74 58.7,18.64 59,18.94 IC4.3 | 50.45,14.79 51,14.24 U1.48 51.1,14.14 51.1,13.74 U1.47 51,13.64 50.2,13.64 50.2,10.64 | 50.45,14.79 49.8,15.44 U1.1 | U1.42 51.1,11.14 51.1,10.74 U1.41 51,10.64 50.2,10.64 | 50.2,8.94 50.2,7.74 49.8,7.34 U1.36 | 50.2,8.94 50.4,9.14 51,9.14 U1.38 | 50.2,8.94 50.2,10.64 | U20.2 67.3,19.04 66.5,19.04 v66.5,17.24 66.5,15.64 67.7,14.44 67.7,13.64 68.3,13.04 68.6,13.04 IC3.1 | C50.1 19.6,7.54 18.9,6.84 v18.9,6.44 18.9,5.14 C52.- 18.9,5.04 18.9,2.54 C53.+ | C64.- 46,3.84 v47.7,3.84 49.3,3.84 C62.- | C51.1 v32.4,22.24 C49.1 | 79.4,11.44 79.4,12.64 C55.2 | 79.4,11.44 79.4,10.24 C54.2 | C65.1 55.2,8.94 v55.2,10.14 55.2,11.34 C66.1 | v23.7,7.64 24.7,7.64 C48.1 | v24.8,11.64 24.8,12.64 C47.1 | v56.5,15.04 56.5,14.04 C63.2 | v60.3,15.44 60.3,16.44 C71.1 | v67.4,8.94 68.6,8.94 U21.2 | v79.6,11.44 79.4,11.44 | v50.5,14.94 50.5,14.84 50.45,14.79
AGND2  (via drill 0.61)  (1 unrouted)
  Top 0.254: R83.2 73.1,50.8 v74.2,51.9 74.3,52 74.3,53.3 R17.2.2 74.2,53.4 73.7,53.9 73.7,60.2 73.75,60.25 | 73.75,60.25 73.7,60.3 73.7,64.1 74.3,64.7 R60.2 | 73.75,60.25 C100.2 | 60.3,58 60.3,59.6 C103.2 | 60.3,58 60.3,57.2 C102.1 | 60.3,58 v58.7,58 58.7,66.9 59,67.2 IC6.3 | 50.45,63.05 51,62.5 U25.48 51.1,62.4 51.1,62 U25.47 51,61.9 50.2,61.9 50.2,58.9 | 50.45,63.05 49.8,63.7 U25.1 | U25.42 51.1,59.4 51.1,59 U25.41 51,58.9 50.2,58.9 | 50.2,57.2 50.2,56 49.8,55.6 U25.36 | 50.2,57.2 50.4,57.4 51,57.4 U25.38 | 50.2,57.2 50.2,58.9 | U32.2 67.3,67.3 66.5,67.3 v66.5,65.5 66.5,63.9 67.7,62.7 67.7,61.9 68.3,61.3 68.6,61.3 IC5.1 | C92.1 19.6,55.8 18.9,55.1 v18.9,54.7 18.9,53.4 C94.- 18.9,53.3 18.9,50.8 C95.+ | C106.- 46,52.1 v47.7,52.1 49.3,52.1 C104.- | C93.1 v32.4,70.5 C91.1 | 79.4,59.7 79.4,60.9 C97.2 | 79.4,59.7 79.4,58.5 C96.2 | C107.1 55.2,57.2 v55.2,58.4 55.2,59.6 C108.1 | v23.7,55.9 24.7,55.9 C90.1 | v24.8,59.9 24.8,60.9 C89.1 | v56.5,63.3 56.5,62.3 C105.2 | v60.3,63.7 60.3,64.7 C113.1 | v67.4,57.2 68.6,57.2 U33.2 | v79.6,59.7 79.4,59.7 | v50.5,63.2 50.5,63.1 50.45,63.05
AGND3  (via drill 0.61)  (1 unrouted)
  Top 0.254: R111.2 73.1,26.67 v74.2,27.77 74.3,27.87 74.3,29.17 R17.3.2 74.2,29.27 73.7,29.77 73.7,36.07 73.75,36.12 | 73.75,36.12 73.7,36.17 73.7,39.97 74.3,40.57 R88.2 | 73.75,36.12 C142.2 | 60.3,33.87 60.3,35.47 C145.2 | 60.3,33.87 60.3,33.07 C144.1 | 60.3,33.87 v58.7,33.87 58.7,42.77 59,43.07 IC8.3 | 50.45,38.92 51,38.37 U37.48 51.1,38.27 51.1,37.87 U37.47 51,37.77 50.2,37.77 50.2,34.77 | 50.45,38.92 49.8,39.57 U37.1 | U37.42 51.1,35.27 51.1,34.87 U37.41 51,34.77 50.2,34.77 | 50.2,33.07 50.2,31.87 49.8,31.47 U37.36 | 50.2,33.07 50.4,33.27 51,33.27 U37.38 | 50.2,33.07 50.2,34.77 | U44.2 67.3,43.17 66.5,43.17 v66.5,41.37 66.5,39.77 67.7,38.57 67.7,37.77 68.3,37.17 68.6,37.17 IC7.1 | C134.1 19.6,31.67 18.9,30.97 v18.9,30.57 18.9,29.27 C136.- 18.9,29.17 18.9,26.67 C137.+ | C148.- 46,27.97 v47.7,27.97 49.3,27.97 C146.- | C135.1 v32.4,46.37 C133.1 | 79.4,35.57 79.4,36.77 C139.2 | 79.4,35.57 79.4,34.37 C138.2 | C149.1 55.2,33.07 v55.2,34.27 55.2,35.47 C150.1 | v23.7,31.77 24.7,31.77 C132.1 | v24.8,35.77 24.8,36.77 C131.1 | v56.5,39.17 56.5,38.17 C147.2 | v60.3,39.57 60.3,40.57 C155.1 | v67.4,33.07 68.6,33.07 U45.2 | v79.6,35.57 79.4,35.57 | v50.5,39.07 50.5,38.97 50.45,38.92
GNDI  (15 unrouted)
  Top 0.254: 42.9,86.13 U6.14 42.9,86.13
  pour Top: -2.54,101.6 91.44,101.6 90.17,-1.27 -3.81,-1.27
  pour top_internal: -3.81,102.87 91.44,102.87 90.17,-1.27 -5.08,-1.27
GNDI1  (15 unrouted)
  Top 0.254: 42.9,13.74 U1.14 42.9,13.74
GNDI2  (15 unrouted)
  Top 0.254: 42.9,62 U25.14 42.9,62
GNDI3  (15 unrouted)
  Top 0.254: 42.9,37.87 U37.14 42.9,37.87
ISOL_GND  (via drill 0.61)
  Top 0.254: 113.5,84.13 113.5,87.13 112.4,88.23 111.9,88.23 U14.4 | 113.5,84.13 113.5,78.93 114.9,77.53 C41.1 | 104.75,80.08 105,80.33 U15.2 105.1,80.43 105.1,80.93 U15.1 105,81.03 105,83.63 | 104.75,80.08 104.1,79.43 104.1,77.83 105,77.83 U15.6 | U15.3 105,79.73 104.8,79.93 104.8,80.03 104.75,80.08 | 105,83.63 102.3,86.33 R25.2 | U12.4 95.4,79.43 95.4,83.13 U11.5 95.2,83.23 92.8,83.23 92.8,92.33 95.3,94.83 95.3,94.93 | 102.7,94.93 102.7,97.73 C37.- | 102.7,94.93 102.7,94.03 C38.- | v112.1,77.13 110.9,77.13 U15.10 | 116.7,93.73 116.7,93.43 117.4,92.73 C42.1 | 116.7,93.73 116.7,94.33 | 116.7,94.33 116.7,97.23 116.2,97.73 C39.1 | 116.7,94.33 113.6,94.33 113.4,94.53 113.4,94.83 113.1,95.13 U13.2 113,95.33 113,95.53 112.4,96.13 111.3,96.13 109.8,97.63 C40.1 109.8,97.73 108.8,96.73 108.8,94.23 108.6,94.03 C35.2 108.6,93.93 108.6,91.53 C36.2 108.5,91.33 108.5,83.63 105,83.63 | v116.8,93.73 116.7,93.73 | 95.3,94.93 102.7,94.93 | 95.3,94.93 95.3,96.43 U10.P$2 | v113.6,84.13 113.5,84.13
  pour Bottom: 93.98,100.33 220.98,100.33 220.98,-1.27 93.98,-1.27
ISOL_GND1  (via drill 0.61)
  Top 0.254: 113.5,11.74 113.5,14.74 112.4,15.84 111.9,15.84 U18.4 | 113.5,11.74 113.5,6.54 114.9,5.14 C80.1 | 104.75,7.69 105,7.94 U17.2 105.1,8.04 105.1,8.54 U17.1 105,8.64 105,11.24 | 104.75,7.69 104.1,7.04 104.1,5.44 105,5.44 U17.6 | U17.3 105,7.34 104.8,7.54 104.8,7.64 104.75,7.69 | 105,11.24 102.3,13.94 R54.2 | U16.4 95.4,7.04 95.4,10.74 U3.5 95.2,10.84 92.8,10.84 92.8,19.94 95.3,22.44 95.3,22.54 | 102.7,22.54 102.7,25.34 C83.- | 102.7,22.54 102.7,21.64 C84.- | v112.1,4.74 110.9,4.74 U17.10 | 116.7,21.34 116.7,21.04 117.4,20.34 C79.1 | 116.7,21.34 116.7,21.94 | 116.7,21.94 116.7,24.84 116.2,25.34 C82.1 | 116.7,21.94 113.6,21.94 113.4,22.14 113.4,22.44 113.1,22.74 U19.2 113,22.94 113,23.14 112.4,23.74 111.3,23.74 109.8,25.24 C81.1 109.8,25.34 108.8,24.34 108.8,21.84 108.6,21.64 C76.2 108.6,21.54 108.6,19.14 C75.2 108.5,18.94 108.5,11.24 105,11.24 | v116.8,21.34 116.7,21.34 | 95.3,22.54 102.7,22.54 | 95.3,22.54 95.3,24.04 U24.P$2 | v113.6,11.74 113.5,11.74
ISOL_GND2  (via drill 0.61)
  Top 0.254: 113.5,60 113.5,63 112.4,64.1 111.9,64.1 U30.4 | 113.5,60 113.5,54.8 114.9,53.4 C122.1 | 104.75,55.95 105,56.2 U29.2 105.1,56.3 105.1,56.8 U29.1 105,56.9 105,59.5 | 104.75,55.95 104.1,55.3 104.1,53.7 105,53.7 U29.6 | U29.3 105,55.6 104.8,55.8 104.8,55.9 104.75,55.95 | 105,59.5 102.3,62.2 R82.2 | U28.4 95.4,55.3 95.4,59 U27.5 95.2,59.1 92.8,59.1 92.8,68.2 95.3,70.7 95.3,70.8 | 102.7,70.8 102.7,73.6 C125.- | 102.7,70.8 102.7,69.9 C126.- | v112.1,53 110.9,53 U29.10 | 116.7,69.6 116.7,69.3 117.4,68.6 C121.1 | 116.7,69.6 116.7,70.2 | 116.7,70.2 116.7,73.1 116.2,73.6 C124.1 | 116.7,70.2 113.6,70.2 113.4,70.4 113.4,70.7 113.1,71 U31.2 113,71.2 113,71.4 112.4,72 111.3,72 109.8,73.5 C123.1 109.8,73.6 108.8,72.6 108.8,70.1 108.6,69.9 C118.2 108.6,69.8 108.6,67.4 C117.2 108.5,67.2 108.5,59.5 105,59.5 | v116.8,69.6 116.7,69.6 | 95.3,70.8 102.7,70.8 | 95.3,70.8 95.3,72.3 U36.P$2 | v113.6,60 113.5,60
ISOL_GND3  (via drill 0.61)
  Top 0.254: 113.5,35.87 113.5,38.87 112.4,39.97 111.9,39.97 U42.4 | 113.5,35.87 113.5,30.67 114.9,29.27 C164.1 | 104.75,31.82 105,32.07 U41.2 105.1,32.17 105.1,32.67 U41.1 105,32.77 105,35.37 | 104.75,31.82 104.1,31.17 104.1,29.57 105,29.57 U41.6 | U41.3 105,31.47 104.8,31.67 104.8,31.77 104.75,31.82 | 105,35.37 102.3,38.07 R110.2 | U40.4 95.4,31.17 95.4,34.87 U39.5 95.2,34.97 92.8,34.97 92.8,44.07 95.3,46.57 95.3,46.67 | 102.7,46.67 102.7,49.47 C167.- | 102.7,46.67 102.7,45.77 C168.- | v112.1,28.87 110.9,28.87 U41.10 | 116.7,45.47 116.7,45.17 117.4,44.47 C163.1 | 116.7,45.47 116.7,46.07 | 116.7,46.07 116.7,48.97 116.2,49.47 C166.1 | 116.7,46.07 113.6,46.07 113.4,46.27 113.4,46.57 113.1,46.87 U43.2 113,47.07 113,47.27 112.4,47.87 111.3,47.87 109.8,49.37 C165.1 109.8,49.47 108.8,48.47 108.8,45.97 108.6,45.77 C160.2 108.6,45.67 108.6,43.27 C159.2 108.5,43.07 108.5,35.37 105,35.37 | v116.8,45.47 116.7,45.47 | 95.3,46.67 102.7,46.67 | 95.3,46.67 95.3,48.17 U48.P$2 | v113.6,35.87 113.5,35.87
N$1
  Top 0.254: R6.2 4.4,74.93 3.2,76.13 3.2,77.43 C3.1 3.2,77.53 3.2,79.13 5.3,81.23 L1.2
N$2
  Top 0.254: R2.1 3.2,88.83 3.2,85.13 C1.1 3.1,85.03 3.1,82.03 2.4,81.33 L1.1
N$3
  Top 0.254: C3.2 4.5,77.43 9.5,77.43 R7.2 9.6,77.53 9.6,79.23 11.6,81.23 L2.2
N$4
  Top 0.254: C1.2 4.5,85.13 8.2,85.13 R3.1 8.3,85.03 8.3,81.63 8.6,81.33 L2.1
N$5
  Top 0.254: 14.6,74.23 16.4,74.23 16.5,74.33 16.5,83.53 18.8,83.53 U$1.11 | 14.6,74.23 R9.1 14.6,75.03 14.6,77.43 R11.2 14.6,77.53 14.6,81.23 C9.1 | 14.6,74.23 3.9,74.23 3.2,74.93 R6.1
N$6  (via drill 0.61, 0.61 layers 1-2)
  Top 0.254: R8.1 10.8,77.43 R7.1 10.9,77.53 v13.7,80.33 | 23.8,83.53 24.2,83.53 24.2,83.13 24.7,82.63 R12.2 | 23.8,83.53 21.8,83.53 U$1.2 | v31.9,88.13 31.9,89.63 32.4,90.13 C10.1 | 23.8,83.53 v23.8,83.23
  top_internal 0.254: v13.7,80.33 16.6,83.23 v23.8,83.23
  bottom_internal 0.254: v31.9,88.13 27,83.23 v23.8,83.23
N$7
  Top 0.254: R20.2 24.8,76.13 25.5,75.43 29.8,75.43 29.8,76.13 U9.1
N$8
  Top 0.254: X1.3 16.5,90.13 14.8,88.43 14.8,86.53 13.4,85.13 R1.2 13.3,85.03 13.3,84.33 9.1,84.33 8.9,84.53 8.9,85.83 7.5,85.83 4.5,88.83 R2.2
N$9
  Top 0.254: R3.2 9.6,85.13 12,85.13 R1.1 12,85.23 14.4,87.63 14.4,89.13 15.5,90.23 15.5,91.63 16.5,92.63 X1.4
N$10
  Top 0.254: R11.1 15.9,77.53 15.9,81.23 C9.2 15.9,81.33 15.9,84.13 | 15.9,84.13 18.8,84.13 U$1.10 | 15.9,84.13 15.9,85.03 R14.2
N$11  (via drill 0.61 layers 1-2)
  Top 0.254: C10.2 31.1,87.23 | 31.1,87.23 R15.2 | 26.7,86.93 25,86.93 24,85.93 24,84.03 21.8,84.03 U$1.3 | 26.7,86.93 26.7,84.53 26.1,83.93 26.1,82.63 R12.1 | v30.3,87.23 31.1,87.23 | v28.3,87.13 26.7,87.13 26.7,86.93
  top_internal 0.254: v30.3,87.23 30.2,87.13 v28.3,87.13
N$12  (via drill 0.61 layers 1-2)
  Top 0.254: R14.1 18,85.93 v18,86.13 | v25.3,86.13 26,85.43 26,85.13 C11.2 | v52.3,82.03 51.1,82.03 U6.39
  top_internal 0.254: v18,86.13 v25.3,86.13 26.1,86.13 28.8,83.43 50.9,83.43 v52.3,82.03
N$13  (via drill 0.61)
  Top 0.254: R15.1 32.4,85.03 | 32.4,85.03 32.4,83.13 31.8,82.53 31.8,79.93 26.1,79.93 C12.2 | v52.3,83.23 52.3,84.03 51.1,84.03 U6.43 | 32.4,85.03 v38.6,85.03
  bottom_internal 0.254: v52.3,83.23 50.5,85.03 v38.6,85.03
N$16  (via drill 0.61 layers 1-2)
  Top 0.254: X1.9 24.1,90.23 24.1,92.63 X1.10 | U10.P$7 82.5,96.43 79.8,93.73 73.4,93.73 73.4,92.83 C2..- 73.4,92.63 72.2,91.43 72.2,87.33 69.6,87.33 69.5,87.23 68.8,87.23 IC1.3 68.7,87.23 68.7,86.43 IC1.2 68.8,86.43 69.5,85.73 69.5,84.43 v62.6,84.43
  top_internal 0.254: v62.6,84.43 58.4,84.43 53.9,88.93 25.4,88.93 24.2,90.13 X1.9
N$17  (via drill 0.61 layers 1-2)
  Top 0.254: v74.9,85.23 74.9,82.33 77.4,82.33 77.6,82.53 78,82.53 C17.1 | v66.8,93.33 64.8,93.33 64.8,92.43 U4.4
  top_internal 0.254: v66.8,93.33 v74.9,85.23
N$18  (via drill 0.61 layers 1-2)
  Top 0.254: X1.7 21.6,90.23 21.6,92.63 X1.8 21.7,92.73 26.6,97.63 v48.5,97.63 | U7.1 68.7,75.33 69.5,75.33 69.5,76.53 68.9,77.13 68.7,77.13 U7.3 68.7,77.23 68.7,80.33 U5.1 68.8,80.23 69.5,80.93 69.5,82.23 | 69.5,82.23 U5.3 | 68.2,90.53 67.4,90.53 U4.1 | 68.2,90.53 68.2,91.83 67.7,92.33 67.4,92.33 U4.3 67.7,92.43 67.7,94.83 | 67.7,94.83 67.7,95.23 67.4,95.53 U8.1 67.6,95.43 68.2,96.03 68.2,96.53 | 68.2,96.53 68.2,97.43 67.4,97.43 U8.3 | 68.2,96.53 73.4,96.53 C25.+ 73.5,96.63 73.5,98.13 83.4,98.13 85,96.53 U10.P$6 | v69.9,86.53 69.9,82.73 69.5,82.33 69.5,82.23 | v69.9,88.13 68.2,89.83 68.2,90.53 | 67.7,94.83 v60.4,94.83
  top_internal 0.254: v69.9,88.13 v69.9,86.53 | v48.5,97.63 51,95.13 60.1,95.13 v60.4,94.83
N$20  (via drill 0.61 layers 1-2)
  Top 0.254: v77.1,83.13 77.1,84.13 78,85.03 C19.1 | v67.6,83.03 66.1,83.03 66.1,82.23 U5.4
  top_internal 0.254: v77.1,83.13 77,83.03 v67.6,83.03
N$22
  Top 0.254: X3.10 24.1,44.43 24.1,41.93 X3.9 24.2,41.83 24.2,20.43 X4.10 | 24.2,44.53 X3.10 | 24.2,44.63 X3.10 | 24.2,44.73 X3.10 | X2.10 24.1,68.53 24.1,66.13 X2.9 24.2,65.93 24.2,44.83 X3.10
N$23
  Top 0.254: C31.1 49,96.53 49.3,96.83 49.3,98.13 49.5,98.33 64.7,98.33 64.7,97.53 U8.4
N$24
  Top 0.254: X4.7 21.6,17.83 21.6,20.23 X4.8 21.6,20.43 21.6,41.83 X3.7 21.6,41.93 21.6,44.43 X3.8 | 21.6,44.53 X3.8 | 21.6,44.63 X3.8 | 21.6,44.73 X3.8 | X2.8 21.6,68.53 21.6,66.13 X2.7 21.6,65.93 21.6,44.83 X3.8
N$26
  Top 0.254: C26.1 73,81.23 69.9,78.13 69.9,75.13 69.5,74.73 65.1,74.73 65.1,76.23 66,77.13 U7.4
N$27  (via drill 0.61 layers 1-2)
  Top 0.254: v60.7,85.23 60.7,86.03 60.4,86.33 R5.1 | v62.6,86.23 66,86.23 66,87.23 IC1.4 | v70.7,85.63 71.1,85.63 72.6,87.13 72.6,88.43 73,88.83 R4.1
  top_internal 0.254: v60.7,85.23 61.7,86.23 v62.6,86.23 67.4,86.23 67.9,85.73 70.6,85.73 v70.7,85.63
N$28  (via drill 0.61 layers 1-2)
  Top 0.254: IC2.6 59,96.63 57.8,96.63 IC2.7 58,96.53 58,94.03 57.1,93.13 50.8,93.13 v50.3,92.63 | v18.8,85.33 18.8,84.63 U$1.9 | v21.9,85.33 21.8,85.23 21.8,84.63 U$1.4 | 30.55,92.08 30.5,92.03 30.5,88.53 29.5,87.53 29.5,85.63 v27.5,83.63 | 30.55,92.08 31.1,92.63 C43.2 | v37.9,92.53 33,92.53 33,92.13 32.9,92.03 30.6,92.03 30.55,92.08
  top_internal 0.254: v18.8,85.33 v21.9,85.33 22,85.33 22.3,85.63 23.3,85.63 23.6,85.33 25.8,85.33 v27.5,83.63 | v50.3,92.63 50.2,92.53 v37.9,92.53
N$30  (via drill 0.61 layers 1-2)
  Top 0.254: v56.6,75.13 56.6,76.13 R16.2 | v58.2,75.13 61.6,75.13 61.6,76.13 R13.1 61.7,76.23 61.7,76.63 62.2,77.13 62.2,82.73 | C13.1 62.2,83.23 62.2,82.73 | v59.5,82.93 59.5,88.13 59.6,88.23 59.6,95.83 60.3,96.53 IC2.5 | 62.2,82.73 v61.8,82.73
  top_internal 0.254: v58.2,75.13 v56.6,75.13 | v59.5,82.93 59.7,82.73 v61.8,82.73
N$31  (via drill 0.61 layers 1-2)
  Top 0.254: v33,79.23 29.1,79.23 26.1,76.23 R20.1 | v34.6,80.83 37,83.23 42,83.23 42,82.33 42.2,82.13 42.8,82.13 U6.22
  top_internal 0.254: v34.6,80.83 v33,79.23
N$32
  Top 0.254: R16.1 55.2,76.23 52.3,76.23 C20.+ 52.3,79.83 51.1,81.03 U6.37
N$33
  Top 0.254: C21.1 55.2,86.33 52,86.33 52,85.83 51.8,85.63 51.1,85.63 U6.46
N$34  (via drill 0.61 layers 1-2)
  Top 0.254: v109.6,77.73 110.8,77.73 U15.11
  top_internal 0.254: v109.6,77.73 110.3,78.43 122.9,78.43 124.4,79.93 X5.1
N$35  (via drill 0.61 layers 1-2)
  Top 0.254: v112.3,79.23 112.3,78.43 110.9,78.43 U15.12
  top_internal 0.254: v112.3,79.23 113,79.93 121.9,79.93 X5.2
N$36
  Top 0.254: R19.1 38.8,82.53 39.7,81.63 42.8,81.63 U6.23
N$37
  Top 0.254: 36.8,79.93 36.8,81.93 37.4,82.53 R19.2 | 36.8,79.93 36.8,76.83 37.4,76.23 R18.2 | 36.8,79.93 33.3,79.93 33.1,80.13 33.1,80.63 32.4,81.33 U9.6
N$38
  Top 0.254: R18.1 38.8,76.23 39,76.43 39,77.33 40.5,78.83 46.2,78.83 46.2,79.63 U6.29
N$39
  Top 0.254: U9.2 31.2,76.23 32.3,76.23 U9.3
N$40  (via drill 0.61 layers 1-2)
  Top 0.254: R10.2 56.5,91.33 IC2.1 56.4,90.73 52.2,90.73 51.5,91.43 C8.1 51.3,91.43 v49.9,91.43 | 15.2,83.23 15.3,83.23 15.3,75.43 15.8,74.93 R9.2 | 15.2,83.23 14.2,83.23 13.6,82.63 13.6,81.43 10.2,78.03 10.2,75.53 9.6,74.93 R8.2 | v27.3,91.73 22.5,86.93 15.2,86.93 15.2,83.23
  top_internal 0.254: v49.9,91.43 49.6,91.73 v27.3,91.73
N$41
  Top 0.254: C8.2 52.8,91.53 55.9,91.53 55.9,92.53 56.1,92.73 57.7,92.73 57.7,91.43 IC2.2 57.8,91.33 R10.1 57.8,78.73 60.3,76.23 R13.2
N$42  (via drill 0.61 layers 1-2)
  Top 0.254: v40.6,84.23 36.5,84.23 33.7,81.43 U9.5 | v75.3,81.53 78.8,81.53 78.8,85.63 79,85.83 90.1,85.83 U11.2
  top_internal 0.254: v40.6,84.23 40.8,84.03 61.9,84.03 63.8,82.13 74.7,82.13 v75.3,81.53
N$43
  Top 0.254: R21.1 38.8,78.83 39.9,78.83 41.7,80.63 43.8,80.63 43.8,82.33 43.6,82.53 42.9,82.53 U6.21
N$44  (via drill 0.61 layers 1-2)
  Top 0.254: v38,79.83 38,79.33 37.5,78.83 R21.2 | v74.5,79.83 78.5,79.83 80.6,81.93 88.7,81.93 88.7,83.53 89.6,84.43 90.1,84.43 U11.3
  top_internal 0.254: v74.5,79.83 v38,79.83
N$45  (via drill 0.61 layers 1-2)
  Top 0.254: 55.9,77.33 55.9,75.73 55.4,75.23 50.7,75.23 50.7,78.13 50,78.83 49.3,78.83 49.3,79.63 U6.35 | 55.9,77.33 55.9,78.13 56.5,78.73 C24.2 | v75.3,78.03 78.6,78.03 79.3,78.73 R17.2 | 55.9,77.33 v56.6,77.33
  top_internal 0.254: v75.3,78.03 74.6,77.33 v56.6,77.33
N$46
  Top 0.254: R17.1 78.1,78.83 78.8,79.53 88.7,79.53 88.7,79.03 89.6,78.13 90.1,78.13 U12.6
N$47  (via drill 0.61 layers 1-2)
  Top 0.254: v48.3,78.23 48.7,78.63 48.7,79.63 U6.34 | v63,76.23 65,74.23 88.7,74.23 88.7,75.93 89.6,76.83 U12.7
  top_internal 0.254: v48.3,78.23 50.3,76.23 v63,76.23
N$50
  Top 0.254: 113.1,78.03 116.2,74.93 R27.1 | 113.1,78.03 113.1,83.23 111.9,84.43 U14.1 | U12.3 95.3,78.03 93.9,78.03 93.9,75.23 94.4,74.73 113,74.73 113,78.03 113.1,78.03
N$51  (via drill 0.61 layers 1-2)
  Top 0.254: v103.8,80.93 103.8,82.33 99.8,86.33 R24.2 | v106.3,78.43 105.1,78.43 U15.5
  top_internal 0.254: v106.3,78.43 v103.8,80.93
N$52
  Top 0.254: R23.2 103.7,79.83 103.7,77.63 104.2,77.13 105,77.13 U15.7
N$53  (via drill 0.61 layers 1-2)
  Top 0.254: v98.4,85.23 98.4,86.33 R24.1 | v93.6,85.23 95.3,85.23 95.3,85.63 U11.7
  top_internal 0.254: v93.6,85.23 v98.4,85.23
N$54  (via drill 0.61 layers 1-2)
  Top 0.254: v98.4,82.73 98.4,83.73 R23.1 | v96.8,82.33 96.7,82.43 96.7,83.53 95.8,84.43 95.4,84.43 U11.6
  top_internal 0.254: v98.4,82.73 98,82.33 v96.8,82.33
N$55  (via drill 0.61 layers 1-2)
  Top 0.254: v109.6,78.93 109.6,79.03 110.8,79.03 U15.13
  top_internal 0.254: v109.6,78.93 112.2,81.53 123.4,81.53 124.4,82.53 X5.3
N$56  (via drill 0.61 layers 1-2)
  Top 0.254: v113.8,74.93 R27.2 | v112.1,75.73 111.4,76.43 110.9,76.43 U15.9
  top_internal 0.254: v113.8,74.93 113,75.73 v112.1,75.73
N$57  (via drill 0.61 layers 1-2)
  Top 0.254: v107.1,91.43 103.6,91.43 R26.1 | v96.8,80.23 96.8,76.93 95.4,76.93 U12.2
  top_internal 0.254: 107.65,90.88 110.9,87.63 X5.8 | 107.65,90.88 v107.1,91.43 | v96.8,80.23 98.5,81.93 98.7,81.93 107.65,90.88
N$58  (via drill 0.61 layers 1-2)
  Top 0.254: v109.3,80.13 109.3,79.73 110.8,79.73 U15.14
  top_internal 0.254: v109.3,80.13 111.7,82.53 121.9,82.53 X5.4
N$59
  Top 0.254: U14.2 111.9,85.73 111.9,86.93 U14.3
N$60  (via drill 0.61)
  Top 0.254: 104.9,86.43 106.6,86.43 106.6,86.93 U14.6 | 104.9,86.43 103.6,86.43 R25.1 | v104.9,86.53 104.9,86.43
  bottom_internal 0.254: v104.9,86.53 124.4,86.53 124.4,87.63 X5.7
N$61  (via drill 0.61 layers 1-2)
  Top 0.254: v100.3,88.33 106.6,88.33 U14.5
  top_internal 0.254: v100.3,88.33 99.8,88.83 97.8,88.83 U10.P$14
N$62  (via drill 0.61 layers 1-2)
  Top 0.254: 107.9,96.73 107.9,88.73 108,88.63 108,85.83 107.25,85.08 | 107.9,96.73 107.9,97.13 108.5,97.73 C40.2 | 107.25,85.08 106.7,84.53 U14.8 | v110.9,97.73 112,97.73 U13.5 | v108,96.73 107.9,96.73 | 107.25,85.08 106.7,85.63 U14.7
  top_internal 0.254: v110.9,97.73 109.9,96.73 v108,96.73
N$63  (via drill 0.61 layers 1-2)
  Top 0.254: v110,83.33 110,80.43 110.8,80.43 U15.15
  top_internal 0.254: v110,83.33 112.8,86.13 123.4,86.13 124.4,85.13 X5.5
N$64  (via drill 0.61 layers 1-2)
  Top 0.254: v117.5,96.73 117.5,97.73 C39.2 | v114.8,96.93 114,97.73 U13.4
  top_internal 0.254: v117.5,96.73 117.3,96.93 v114.8,96.93
N$65  (via drill 0.61)
  Top 0.254: v112.3,80.53 112.3,80.93 110.9,80.93 U15.16
  bottom_internal 0.254: v112.3,80.53 116.8,85.03 121.9,85.03 X5.6
N$66
  Top 0.254: R34.2 4.4,2.54 3.2,3.74 3.2,5.04 C44.1 3.2,5.14 3.2,6.74 5.3,8.84 L3.2
N$67
  Top 0.254: R30.1 3.2,16.44 3.2,12.74 C2.1 3.1,12.64 3.1,9.64 2.4,8.94 L3.1
N$68
  Top 0.254: C44.2 4.5,5.04 9.5,5.04 R35.2 9.6,5.14 9.6,6.84 11.6,8.84 L4.2
N$69
  Top 0.254: C2.2 4.5,12.74 8.2,12.74 R31.1 8.3,12.64 8.3,9.24 8.6,8.94 L4.1
N$70
  Top 0.254: 14.6,1.84 16.4,1.84 16.5,1.94 16.5,11.14 18.8,11.14 U$2.11 | 14.6,1.84 R37.1 14.6,2.64 14.6,5.04 R38.2 14.6,5.14 14.6,8.84 C45.1 | 14.6,1.84 3.9,1.84 3.2,2.54 R34.1
N$71  (via drill 0.61, 0.61 layers 1-2)
  Top 0.254: R36.1 10.8,5.04 R35.1 10.9,5.14 v13.7,7.94 | 23.8,11.14 24.2,11.14 24.2,10.74 24.7,10.24 R39.2 | 23.8,11.14 21.8,11.14 U$2.2 | v31.9,15.74 31.9,17.24 32.4,17.74 C46.1 | 23.8,11.14 v23.8,10.84
  top_internal 0.254: v13.7,7.94 16.6,10.84 v23.8,10.84
  bottom_internal 0.254: v31.9,15.74 27,10.84 v23.8,10.84
N$72
  Top 0.254: X6.3 16.5,17.74 14.8,16.04 14.8,14.14 13.4,12.74 R29.2 13.3,12.64 13.3,11.94 9.1,11.94 8.9,12.14 8.9,13.44 7.5,13.44 4.5,16.44 R30.2
N$73
  Top 0.254: R31.2 9.6,12.74 12,12.74 R29.1 12,12.84 14.4,15.24 14.4,16.74 15.5,17.84 15.5,19.24 16.5,20.24 X6.4
N$74
  Top 0.254: R38.1 15.9,5.14 15.9,8.84 C45.2 15.9,8.94 15.9,11.74 | 15.9,11.74 18.8,11.74 U$2.10 | 15.9,11.74 15.9,12.64 R40.2
N$75  (via drill 0.61 layers 1-2)
  Top 0.254: C46.2 31.1,14.84 | 31.1,14.84 R41.2 | 26.7,14.54 25,14.54 24,13.54 24,11.64 21.8,11.64 U$2.3 | 26.7,14.54 26.7,12.14 26.1,11.54 26.1,10.24 R39.1 | v30.3,14.84 31.1,14.84 | v28.3,14.74 26.7,14.74 26.7,14.54
  top_internal 0.254: v30.3,14.84 30.2,14.74 v28.3,14.74
N$76  (via drill 0.61 layers 1-2)
  Top 0.254: R40.1 18,13.54 v18,13.74 | v25.3,13.74 26,13.04 26,12.74 C47.2 | v52.3,9.64 51.1,9.64 U1.39
  top_internal 0.254: v18,13.74 v25.3,13.74 26.1,13.74 28.8,11.04 50.9,11.04 v52.3,9.64
N$77  (via drill 0.61)
  Top 0.254: R41.1 32.4,12.64 | 32.4,12.64 32.4,10.74 31.8,10.14 31.8,7.54 26.1,7.54 C48.2 | v52.3,10.84 52.3,11.64 51.1,11.64 U1.43 | 32.4,12.64 v38.6,12.64
  bottom_internal 0.254: v52.3,10.84 50.5,12.64 v38.6,12.64
N$78  (via drill 0.61 layers 1-2)
  Top 0.254: v60.7,12.84 60.7,13.64 60.4,13.94 R33.1 | v62.6,13.84 66,13.84 66,14.84 IC3.4 | v70.7,13.24 71.1,13.24 72.6,14.74 72.6,16.04 73,16.44 R32.1
  top_internal 0.254: v60.7,12.84 61.7,13.84 v62.6,13.84 67.4,13.84 67.9,13.34 70.6,13.34 v70.7,13.24
N$79  (via drill 0.61 layers 1-2)
  Top 0.254: IC4.6 59,24.24 57.8,24.24 IC4.7 58,24.14 58,21.64 57.1,20.74 50.8,20.74 v50.3,20.24 | v18.8,12.94 18.8,12.24 U$2.9 | v21.9,12.94 21.8,12.84 21.8,12.24 U$2.4 | 30.55,19.69 30.5,19.64 30.5,16.14 29.5,15.14 29.5,13.24 v27.5,11.24 | 30.55,19.69 31.1,20.24 C49.2 | v37.9,20.14 33,20.14 33,19.74 32.9,19.64 30.6,19.64 30.55,19.69
  top_internal 0.254: v18.8,12.94 v21.9,12.94 22,12.94 22.3,13.24 23.3,13.24 23.6,12.94 25.8,12.94 v27.5,11.24 | v50.3,20.24 50.2,20.14 v37.9,20.14
N$80  (via drill 0.61 layers 1-2)
  Top 0.254: v56.6,2.74 56.6,3.74 R42.2 | v58.2,2.74 61.6,2.74 61.6,3.74 R43.1 61.7,3.84 61.7,4.24 62.2,4.74 62.2,10.34 | C61.1 62.2,10.84 62.2,10.34 | v59.5,10.54 59.5,15.74 59.6,15.84 59.6,23.44 60.3,24.14 IC4.5 | 62.2,10.34 v61.8,10.34
  top_internal 0.254: v58.2,2.74 v56.6,2.74 | v59.5,10.54 59.7,10.34 v61.8,10.34
N$81
  Top 0.254: R42.1 55.2,3.84 52.3,3.84 C62.+ 52.3,7.44 51.1,8.64 U1.37
N$82
  Top 0.254: C63.1 55.2,13.94 52,13.94 52,13.44 51.8,13.24 51.1,13.24 U1.46
N$83  (via drill 0.61 layers 1-2)
  Top 0.254: R44.2 56.5,18.94 IC4.1 56.4,18.34 52.2,18.34 51.5,19.04 C72.1 51.3,19.04 v49.9,19.04 | 15.2,10.84 15.3,10.84 15.3,3.04 15.8,2.54 R37.2 | 15.2,10.84 14.2,10.84 13.6,10.24 13.6,9.04 10.2,5.64 10.2,3.14 9.6,2.54 R36.2 | v27.3,19.34 22.5,14.54 15.2,14.54 15.2,10.84
  top_internal 0.254: v49.9,19.04 49.6,19.34 v27.3,19.34
N$84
